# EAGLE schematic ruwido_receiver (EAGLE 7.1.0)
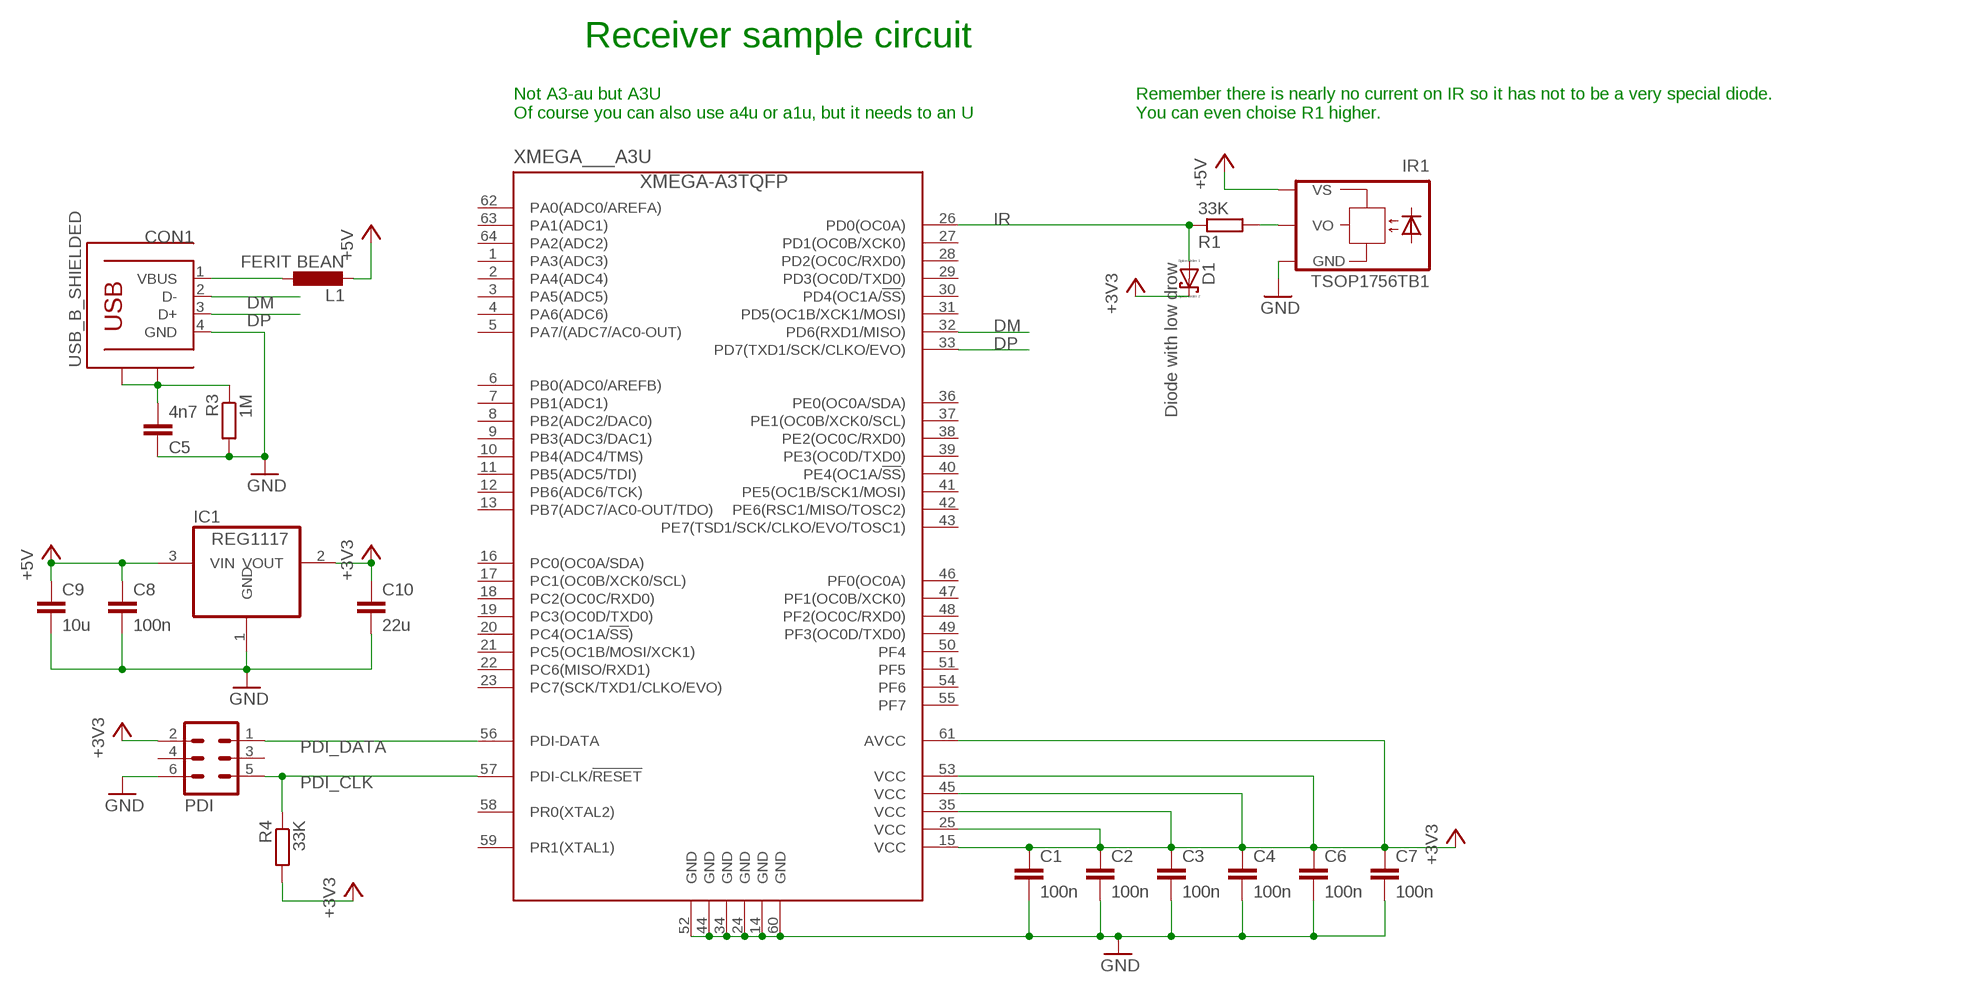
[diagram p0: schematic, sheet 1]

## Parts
C1  100n  C-EUC0603  [C0603]
C2  100n  C-EUC0603  [C0603]
C3  100n  C-EUC0603  [C0603]
C4  100n  C-EUC0603  [C0603]
C5  4n7  C-EU050-050X075  [C050-050X075]
C6  100n  C-EUC0603  [C0603]
C7  100n  C-EUC0603  [C0603]
C8  100n  C-EUC0603  [C0603]
C9  10u  C-EUC0603  [C0603]
C10  22u  C-EUC0603  [C0603]
CON1  USB_B_SHIELDED  [USB_B_SHIELDED_THMD]
D1  Diode with low drow  SCHOTTKY-DIODEDO35-7  [DIODE_DO35-7]
IC1  REG1117  [SOT223]
IR1  TSOP1756TB1  [TSOP17_TB1]
L1  FERIT BEAN  L-EUL2012C  [L2012C]
PDI  ML6  [ML6]
R1  33K  R-EU_R0603  [R0603]
R3  1M  R-EU_0207/10  [0207/10]
R4  33K  R-EU_R0603  [R0603]
XMEGA___A3U  XMEGA-A3TQFP  [TQFP64]

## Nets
+3V3: C1.1 C2.1 C3.1 C4.1 C6.1 C7.1 C10.1 D1.C(A) IC1.2(VOUT) PDI.2 R4.2 XMEGA___A3U.15(VCC) XMEGA___A3U.25(VCC) XMEGA___A3U.35(VCC) XMEGA___A3U.45(VCC) XMEGA___A3U.53(VCC) XMEGA___A3U.61(AVCC)
+5V: C8.1 C9.1 IC1.3(VIN) IR1.VS L1.2
DM: CON1.2(D-) XMEGA___A3U.32(PD6(RXD1/MISO))
DP: CON1.3(D+) XMEGA___A3U.33(PD7(TXD1/SCK/CLKO/EVO))
GND: C1.2 C2.2 C3.2 C4.2 C5.1 C6.2 C7.2 C8.2 C9.2 C10.2 CON1.4(GND) IC1.1(GND) IR1.GND PDI.6 R3.2 XMEGA___A3U.14(GND) XMEGA___A3U.24(GND) XMEGA___A3U.34(GND) XMEGA___A3U.44(GND) XMEGA___A3U.52(GND) XMEGA___A3U.60(GND)
IR: D1.A(C) R1.1 XMEGA___A3U.26(PD0(OC0A))
N$1: IR1.VO R1.2
N$13: C5.2 CON1.S1 CON1.S2 R3.1
PDI_CLK: PDI.5 R4.1 XMEGA___A3U.57(PDI-CLK/!RESET)
PDI_DATA: PDI.1 XMEGA___A3U.56(PDI-DATA)
VBUS: CON1.1(VBUS) L1.1
Unconnected: PDI.3 PDI.4 XMEGA___A3U.1(PA3(ADC3)) XMEGA___A3U.2(PA4(ADC4)) XMEGA___A3U.3(PA5(ADC5)) XMEGA___A3U.4(PA6(ADC6)) XMEGA___A3U.5(PA7/(ADC7/AC0-OUT)) XMEGA___A3U.6(PB0(ADC0/AREFB)) XMEGA___A3U.7(PB1(ADC1)) XMEGA___A3U.8(PB2(ADC2/DAC0)) XMEGA___A3U.9(PB3(ADC3/DAC1)) XMEGA___A3U.10(PB4(ADC4/TMS)) XMEGA___A3U.11(PB5(ADC5/TDI)) XMEGA___A3U.12(PB6(ADC6/TCK)) XMEGA___A3U.13(PB7(ADC7/AC0-OUT/TDO)) XMEGA___A3U.16(PC0(OC0A/SDA)) XMEGA___A3U.17(PC1(OC0B/XCK0/SCL)) XMEGA___A3U.18(PC2(OC0C/RXD0)) XMEGA___A3U.19(PC3(OC0D/TXD0)) XMEGA___A3U.20(PC4(OC1A/!SS!)) XMEGA___A3U.21(PC5(OC1B/MOSI/XCK1)) XMEGA___A3U.22(PC6(MISO/RXD1)) XMEGA___A3U.23(PC7(SCK/TXD1/CLKO/EVO)) XMEGA___A3U.27(PD1(OC0B/XCK0)) XMEGA___A3U.28(PD2(OC0C/RXD0)) XMEGA___A3U.29(PD3(OC0D/TXD0)) XMEGA___A3U.30(PD4(OC1A/!SS!)) XMEGA___A3U.31(PD5(OC1B/XCK1/MOSI)) XMEGA___A3U.36(PE0(OC0A/SDA)) XMEGA___A3U.37(PE1(OC0B/XCK0/SCL)) XMEGA___A3U.38(PE2(OC0C/RXD0)) XMEGA___A3U.39(PE3(OC0D/TXD0)) XMEGA___A3U.40(PE4(OC1A/!SS!)) XMEGA___A3U.41(PE5(OC1B/SCK1/MOSI)) XMEGA___A3U.42(PE6(RSC1/MISO/TOSC2)) XMEGA___A3U.43(PE7(TSD1/SCK/CLKO/EVO/TOSC1)) XMEGA___A3U.46(PF0(OC0A)) XMEGA___A3U.47(PF1(OC0B/XCK0)) XMEGA___A3U.48(PF2(OC0C/RXD0)) XMEGA___A3U.49(PF3(OC0D/TXD0)) XMEGA___A3U.50(PF4) XMEGA___A3U.51(PF5) XMEGA___A3U.54(PF6) XMEGA___A3U.55(PF7) XMEGA___A3U.58(PR0(XTAL2)) XMEGA___A3U.59(PR1(XTAL1)) XMEGA___A3U.62(PA0(ADC0/AREFA)) XMEGA___A3U.63(PA1(ADC1)) XMEGA___A3U.64(PA2(ADC2))

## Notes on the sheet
- Receiver sample circuit
- Not A3-au but A3U
  Of course you can also use a4u or a1u, but it needs to an U
- Remember there is nearly no current on IR so it has not to be a very special diode.
  You can even choise R1 higher.

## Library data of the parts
C1-C4 C6-C10 = rcl:C-EU: CAPACITOR, European symbol
C5 = resistor:C-EU: CAPACITOR, European symbol
CON1 = USB:USB_B_SHIELDED
D1 = eagle-ltspice:SCHOTTKY-DIODE: Schottky Diode; SPICEMODEL: NONE; SPICEPREFIX: D; SPICETYPE: diode
IC1 = burr-brown:REG1117: 800mA and 1A Low Dropout (LDO) Positive Regulator 1.8V, 2.5V, 2.85V, 3.3V, 5V, and Adj; MPN: REG1117; OC_FARNELL: 1097566; OC_NEWARK: 14P6981
IR1 = telefunken:TSOP17*TB1: TSOP17..TB1 IR Receiver Modules for Remote Control Systems Source: http://www.vishay.com/docs/82042/82042.pdf; OC_FARNELL: unknown; OC_NEWARK: unknown
L1 = resistor:L-EU: INDUCTOR, European symbol
PDI = con-harting-ml:ML6: HARTING; OC_FARNELL: unknown; OC_NEWARK: unknown
R1 R4 = rcl:R-EU_: RESISTOR, European symbol
R3 = resistor:R-EU_: RESISTOR, European symbol
XMEGA___A3U = avr-7:XMEGA-A3: Atmel XMega A3 series processor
